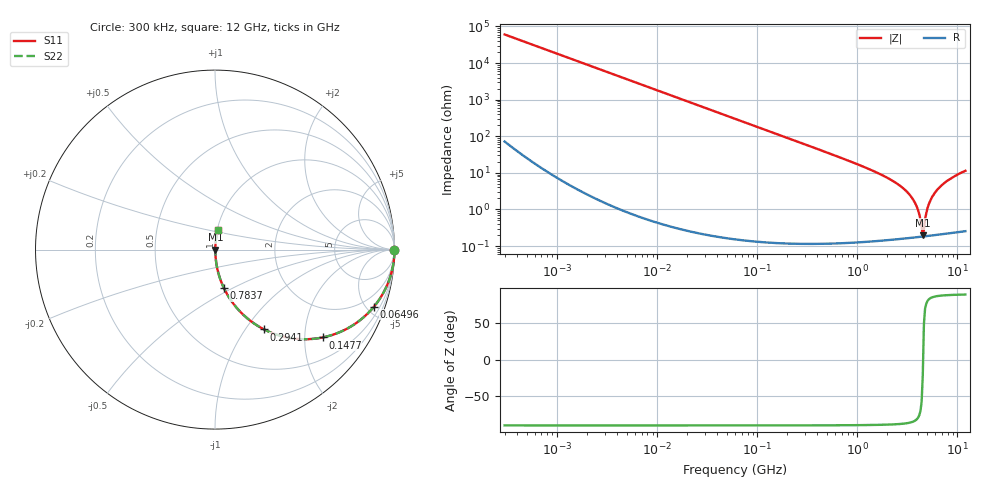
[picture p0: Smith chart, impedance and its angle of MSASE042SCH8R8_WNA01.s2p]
! MSASE042SCH8R8_WNA01  S-PARAMETER MODEL  ( General Type )
! Model Generated by TAIYO YUDEN Corporation (http://www.ty-top.com)
! Version 1.0
! TAIYO YUDEN Control No. 120810
! Copyright(c) 2012 TAIYO YUDEN CO.,LTD. All Rights Reserved.
! Product Description (link to TY-COMPAS)
! https://ds.yuden.co.jp/TYCOMPAS/or/detail?pn=MSASE042SCH8R8BWNA01&u=M
! Products Name : Multilayer Ceramic Capacitors
! Characteristics :
!  Capacitance : 8.8 pF , Rated Voltage : 16V , TCC : CH / C0H
!  Case Size : 0.4 x 0.2 / 0.016 x 0.008 [mm/inch] , Thickness : 0.2 / 0.008 [mm/inch]
!  (Conditions: Temperature = 25 degC , DC Bias Current/Voltage = 0A / 0V)
! External Node Assignments :
!  1  o---| |---o  2
! GND o---------o GND
! Frequency Range : 0.3MHz  -  12000MHz  [ 401 STEP ]
# MHz S RI R 50
! Freq[MHz].  S11 Real  S11 Imag  S21 Real  S21 Imag  S12 Real  S12 Imag  S22 Real  S22 Imag
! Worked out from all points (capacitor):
!   401 points, 300 kHz to 12 GHz, reference 50 ohm
!   read as one part in series: C = 8.8 pF near 316.3 kHz
!   lowest |Z| = 196 mohm at 4.503 GHz (marker M1)
!   series resonance near 4.534 GHz, so ESL is about 140 pH
!   S11 on the Smith chart (normalised r, x): 300 kHz: open; 64.96 MHz: 1.00, -5.57; 147.7 MHz: 1.00, -2.45; 294.1 MHz: 1.00, -1.23; 783.7 MHz: 1.00, -0.45; 12 GHz: 1.01, +0.23
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0.3  1 -0.00166  4.72e-06 0.00166  4.72e-06 0.00166  1 -0.00166
1.769972  0.9999 -0.00978  9.86e-05 0.00978  9.86e-05 0.00978  0.9999 -0.00978
10.44266  0.9967 -0.0575  0.00333 0.0575  0.00333 0.0575  0.9967 -0.0575
26.39317  0.9791 -0.1428  0.0209 0.1428  0.0209 0.1428  0.9791 -0.1428
60  0.9008 -0.2987  0.0992 0.2987  0.0992 0.2987  0.9008 -0.2987
64.96309  0.8856 -0.318  0.1144 0.318  0.1144 0.318  0.8856 -0.318
147.6816  0.5996 -0.4895  0.4004 0.4895  0.4004 0.4895  0.5996 -0.4895
294.0765  0.2733 -0.4447  0.7267 0.4447  0.7267 0.4447  0.2733 -0.4447
353.9943  0.2057 -0.4031  0.7943 0.4031  0.7943 0.4031  0.2057 -0.4031
783.7017  0.0488 -0.2128  0.9512 0.2128  0.9512 0.2128  0.0488 -0.2128
2088.533  0.00609 -0.0678  0.9939 0.0678  0.9939 0.0678  0.00609 -0.0678
2795.104  0.00319 -0.0401  0.9968 0.0401  0.9968 0.0401  0.00319 -0.0401
3454.93  0.00217 -0.022  0.9978 0.022  0.9978 0.022  0.00217 -0.022
3944.255  0.00188 -0.0113  0.9981 0.0113  0.9981 0.0113  0.00188 -0.0113
4385.161  0.00181 -0.00286  0.9982 0.00286  0.9982 0.00286  0.00181 -0.00286
4502.883  0.00182 -0.000721  0.9982 0.000721  0.9982 0.000721  0.00182 -0.000721
4747.894  0.00188 0.00495  0.9981 -0.00495  0.9981 -0.00495  0.00188 0.00495
5006.236  0.00199 0.0104  0.998 -0.0104  0.998 -0.0104  0.00199 0.0104
5278.635  0.00216 0.0158  0.9978 -0.0158  0.9978 -0.0158  0.00216 0.0158
6188.031  0.0031 0.0328  0.9969 -0.0328  0.9969 -0.0328  0.0031 0.0328
8281.503  0.00653 0.0653  0.9935 -0.0653  0.9935 -0.0653  0.00653 0.0653
12000  0.0152 0.1117  0.9848 -0.1117  0.9848 -0.1117  0.0152 0.1117
